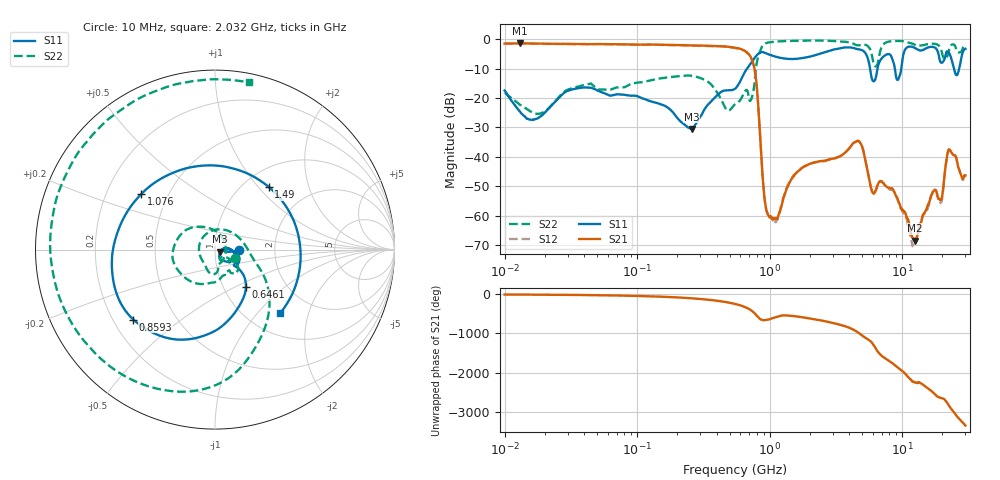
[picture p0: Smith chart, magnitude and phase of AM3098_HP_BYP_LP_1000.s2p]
!Agilent Technologies,E8364B,MY43040894,A.07.50.67
!Agilent E8364B: A.07.50.67
!Date: Wednesday, June 17, 2020 09:20:46
!Correction: S11(Full 2 Port(1,2))
!S21(Full 2 Port(1,2))
!S12(Full 2 Port(1,2))
!S22(Full 2 Port(1,2))
!S2P File: Measurements: S11, S21, S12, S22:Log Frequency Sweep
# Hz S  dB  R 50
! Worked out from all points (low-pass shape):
!   1601 points, 10 MHz to 30 GHz, reference 50 ohm
!   highest |S21| = -1.42 dB at 12.97 MHz (marker M1); lowest = -68.4 dB at 12.56 GHz (marker M2)
!   |S21| within 3 dB of the highest: start of sweep to 670.7 MHz
!   lowest |S11| = -30.5 dB at 258.6 MHz (marker M3), VSWR 1.06, Z = 52.8 - j1.17 ohm
!   |S11| at or under -10 dB: 5.717 GHz to 6.513 GHz (795.8 MHz wide, 13 % of centre); 8.806 GHz to 9.85 GHz (1.045 GHz wide, 11.2 % of centre); 24.62 GHz to 26.94 GHz (2.319 GHz wide, 9 % of centre)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
!   |S22| runs from -25.4 to -0.4 dB; largest |S21 - S12| = 0.015
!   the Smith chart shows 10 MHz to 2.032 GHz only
!   S11 on the Smith chart (normalised r, x): 10 MHz: 1.31, -0.01; 646.1 MHz: 1.27, -0.57; 859.3 MHz: 0.28, -0.34; 1.076 GHz: 0.35, +0.30; 1.49 GHz: 1.28, +1.14; 2.032 GHz: 1.39, -1.33
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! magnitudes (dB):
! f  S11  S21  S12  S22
! 10 MHz  -17.4  -1.5  -1.6  -18.2
! 12.97 MHz  -24.4  -1.4  -1.5  -22.2
! 38.04 MHz  -16.5  -1.7  -1.7  -15.8
! 144.7 MHz  -21.8  -1.9  -1.9  -13.4
! 258.6 MHz  -30.5  -2.2  -2.2  -12.5
! 547.7 MHz  -16.9  -2.9  -3.0  -22.1
! 646.1 MHz  -11.4  -3.9  -4.0  -17.9
! 769.7 MHz  -6.4  -10.2  -10.3  -14.9
! 859.3 MHz  -4.4  -37.7  -37.5  -3.3
! 940.3 MHz  -4.8  -57.8  -57.5  -1.4
! 1.076 GHz  -5.8  -61.1  -61.8  -0.9
! 1.49 GHz  -6.7  -46.9  -47.0  -0.6
! 2.032 GHz  -5.9  -42.3  -42.4  -0.4
! 2.084 GHz  -5.8  -42.1  -42.2  -0.4
! 4.663 GHz  -3.4  -34.5  -34.6  -2.1
! 6.08 GHz  -14.3  -52.4  -52.3  -8.1
! 7.926 GHz  -5.1  -50.4  -50.9  -0.8
! 9.302 GHz  -13.8  -54.8  -54.8  -0.6
! 12.56 GHz  -3.0  -68.4  -68.4  -2.0
! 19.61 GHz  -7.9  -54.7  -55.5  -3.4
! 22.67 GHz  -4.8  -37.4  -37.6  -3.3
! 30 GHz  -3.3  -46.3  -47.0  -2.6
